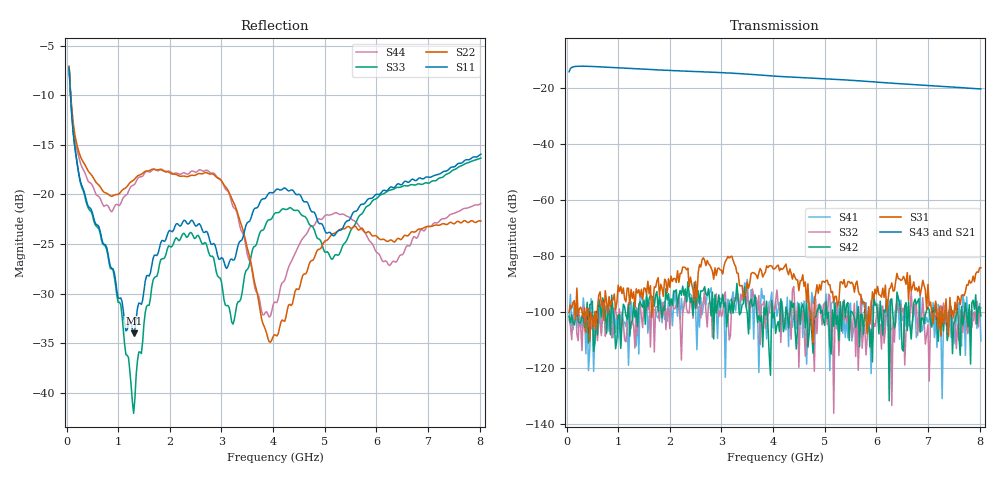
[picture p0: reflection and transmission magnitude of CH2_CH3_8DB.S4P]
!Agilent Technologies,E5071C,MY46316741,A.11.02
!Date: Thu May 28 14:40:17 2026
!Data & Calibration Information:
!1:CH2 INPUT 2:CH2 OUTPUT 3:CH3 INPUT 4:CH3 OUTPUT
!Freq	S11:SOLT4(ON)	S12:SOLT4(ON)	S13:SOLT4(ON)	S14:SOLT4(ON)
!	S21:SOLT4(ON)	S22:SOLT4(ON)	S23:SOLT4(ON)	S24:SOLT4(ON)
!	S31:SOLT4(ON)	S32:SOLT4(ON)	S33:SOLT4(ON)	S34:SOLT4(ON)
!	S41:SOLT4(ON)	S42:SOLT4(ON)	S43:SOLT4(ON)	S44:SOLT4(ON)
!PortZ  Port1:50+j0  Port2:50+j0  Port3:50+j0  Port4:50+j0
!Above PortZ is port z conversion or system Z0 setting when saving the data.
!When reading, reference impedance value at option line is always used.
# Hz S dB R 50
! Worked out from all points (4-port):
!   320 points, 50 MHz to 8.025 GHz, reference 50 ohm
!   strongest paths, dB at 50 MHz, 2.05 GHz, 4.05 GHz, 6.05 GHz, 8.025 GHz:
!     S43: -14.2, -13.8, -15.8, -17.9, -20.3
!     S21: -14.2, -13.8, -16.0, -18.1, -20.5
!     S31: -100.0, -89.0, -84.1, -93.7, -84.0
!     S42: -101.5, -97.5, -107.5, -107.7, -101.3
!     S32: -102.5, -96.9, -96.0, -105.9, -98.4
!     S41: -101.6, -104.8, -95.9, -104.7, -110.2
!   lowest |S11| = -34.0 dB at 1.3 GHz (marker M1), VSWR 1.04, Z = 48.4 - j1.18 ohm
!   |S11| at or under -10 dB: 76.96 MHz to end of sweep
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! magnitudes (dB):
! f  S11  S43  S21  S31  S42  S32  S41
! 50 MHz  -7.2  -14.2  -14.2  -100.0  -101.5  -102.5  -101.6
! 425 MHz  -21.2  -12.3  -12.3  -98.8  -111.0  -103.8  -120.8
! 1.3 GHz  -34.0  -13.1  -13.2  -92.7  -96.5  -104.9  -99.4
! 1.975 GHz  -23.7  -13.7  -13.8  -88.0  -93.4  -98.4  -95.0
! 3.225 GHz  -26.6  -14.7  -14.8  -81.4  -100.3  -97.0  -92.7
! 3.95 GHz  -19.8  -15.6  -15.8  -83.4  -122.4  -96.7  -96.0
! 8.025 GHz  -15.9  -20.3  -20.5  -84.0  -101.3  -98.4  -110.2
